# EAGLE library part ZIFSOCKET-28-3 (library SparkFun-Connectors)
ZIF Socket 28-Pin 0.3" Lever-action ZIF socket for 28-pin ICs SparkFun Products: ZIF Socket 28-Pin
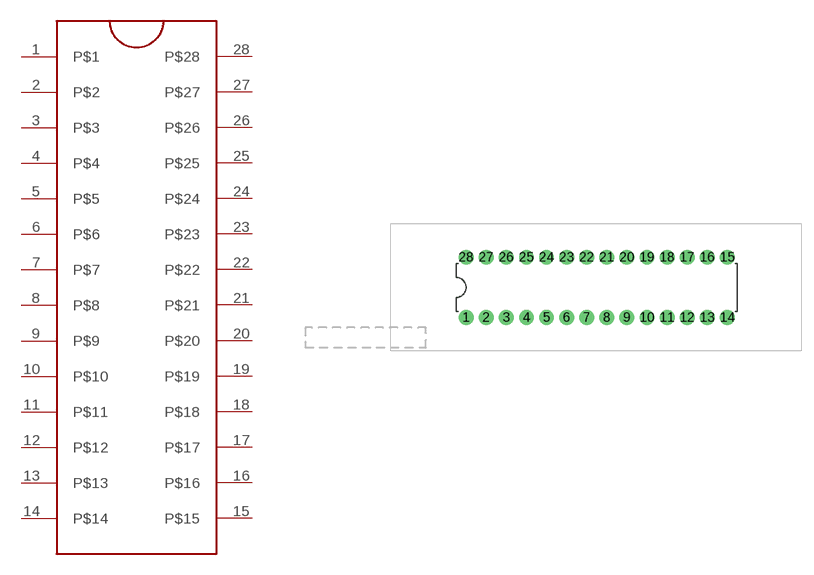
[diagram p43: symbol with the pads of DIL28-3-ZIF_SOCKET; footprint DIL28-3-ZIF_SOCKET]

Designator prefix J

## ZIFSOCKET-28-3" (PROD_ID: CONN-10960; SF_ID: PRT-09175)  [DIL28-3-ZIF_SOCKET]
1  P$1
2  P$2
3  P$3
4  P$4
5  P$5
6  P$6
7  P$7
8  P$8
9  P$9
10  P$10
11  P$11
12  P$12
13  P$13
14  P$14
15  P$15
16  P$16
17  P$17
18  P$18
19  P$19
20  P$20
21  P$21
22  P$22
23  P$23
24  P$24
25  P$25
26  P$26
27  P$27
28  P$28

## Footprint DIL28-3-ZIF_SOCKET (pad centres in mm)
ZIF Socket 28-Pin 0.3" tDocu shows location of lever when unlocked. Specifications: Pin count:28 Example device(s): ZIF_SOCKET_28-3
drill 1.016 pad 1.88: 1 -16.51,-3.81; 2 -13.97,-3.81; 3 -11.43,-3.81; 4 -8.89,-3.81; 5 -6.35,-3.81; 6 -3.81,-3.81; 7 -1.27,-3.81; 8 1.27,-3.81; 9 3.81,-3.81; 10 6.35,-3.81; 11 8.89,-3.81; 12 11.43,-3.81; 13 13.97,-3.81; 14 16.51,-3.81; 15 16.51,3.81; 16 13.97,3.81; 17 11.43,3.81; 18 8.89,3.81; 19 6.35,3.81; 20 3.81,3.81; 21 1.27,3.81; 22 -1.27,3.81; 23 -3.81,3.81; 24 -6.35,3.81; 25 -8.89,3.81; 26 -11.43,3.81; 27 -13.97,3.81; 28 -16.51,3.81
